PROGRAM ACS_SAMPLE_TOGGLE_OUTPUTS
VAR
END_VAR
VAR_IN_OUT 
	Axis:ACS_DRIVE_TYPE;
END_VAR

IF Axis.InputDigitalOutput1 THEN
	Axis.OutputDigitalOutput1 := FALSE;
	Axis.OutputDigitalOutput2 := TRUE;
ELSE
	Axis.OutputDigitalOutput1 := TRUE;
	Axis.OutputDigitalOutput2 := FALSE;		
END_IF

END_PROGRAM
